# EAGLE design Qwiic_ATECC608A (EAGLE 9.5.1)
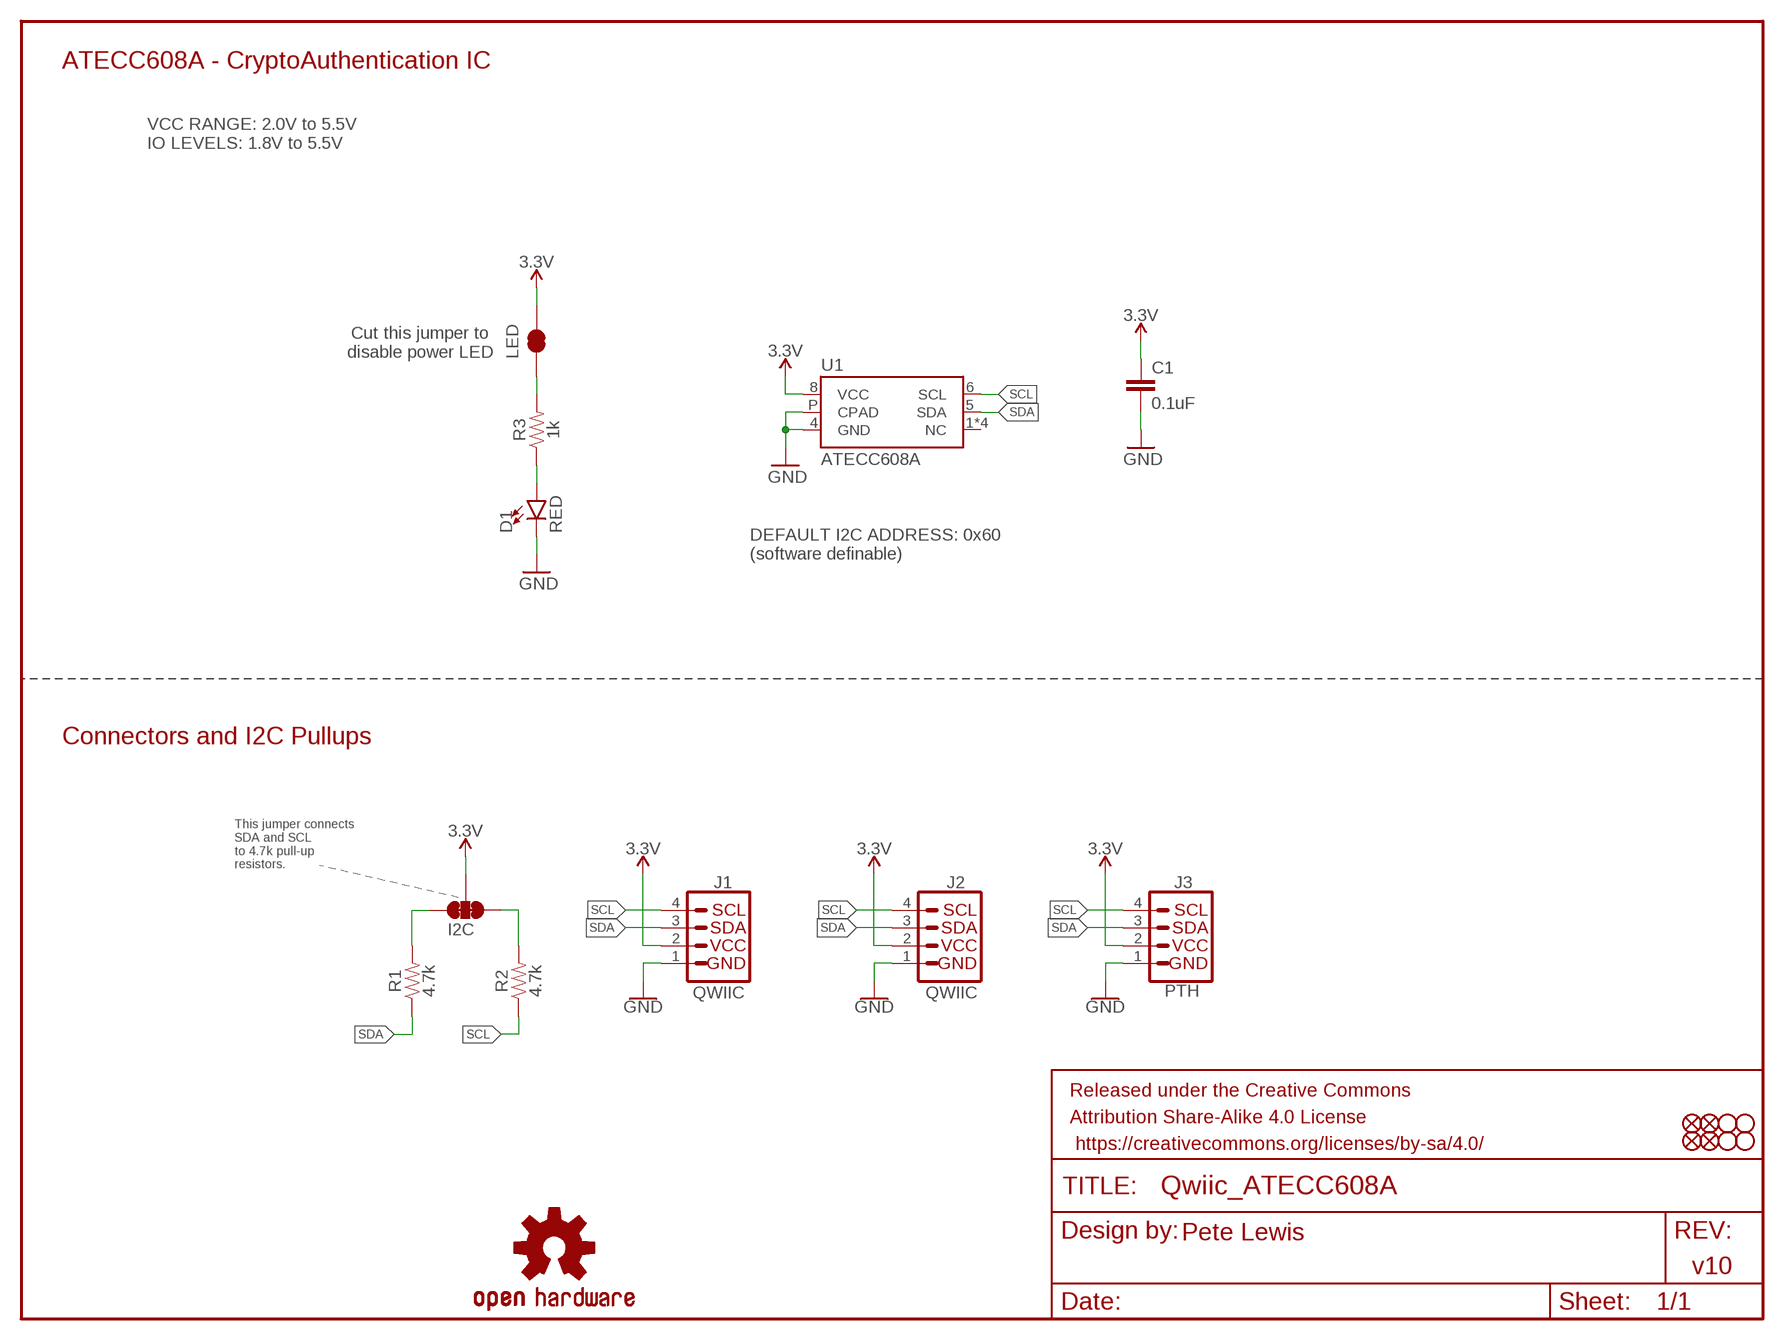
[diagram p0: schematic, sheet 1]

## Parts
C1  0.1uF  0.1UF-0603-25V-(+80/-20%)  [0603]
D1  RED  LED-RED0603  [LED-0603]
FD1  FIDUCIAL1X2  [FIDUCIAL-1X2]
FD2  FIDUCIAL1X2  [FIDUCIAL-1X2]
FD3  FIDUCIAL1X2  [FIDUCIAL-1X2]
FD4  FIDUCIAL1X2  [FIDUCIAL-1X2]
FRAME1  FRAME-LETTER  [CREATIVE_COMMONS]
H1  STAND-OFF  [STAND-OFF]
H2  STAND-OFF  [STAND-OFF]
H3  STAND-OFF  [STAND-OFF]
H4  STAND-OFF  [STAND-OFF]
I2C  JUMPER-SMT_3_2-NC_TRACE_SILK  [SMT-JUMPER_3_2-NC_TRACE_SILK]
J1  QWIIC  I2C_STANDARDQWIIC  [JST04_1MM_RA]
J2  QWIIC  I2C_STANDARDQWIIC  [JST04_1MM_RA]
J3  PTH  I2C_STANDARD_NO_SILK  [1X04_NO_SILK]
LED  JUMPER-SMT_2_NC_TRACE_SILK  [SMT-JUMPER_2_NC_TRACE_SILK]
LOGO4  OSHW-LOGOS  [OSHW-LOGO-S]
R1  4.7k  4.7KOHM-0603-1/10W-1%  [0603]
R2  4.7k  4.7KOHM-0603-1/10W-1%  [0603]
R3  1k  1KOHM-0603-1/10W-1%  [0603]
U1  ATECC608A  ATECC608AUDFN_2X3MM  [UDFN_2X3MM]

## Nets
3.3V: C1.1 I2C.2 J1.2 J2.2 J3.2 LED.2 U1.8(VCC)
GND: C1.2 D1.C J1.1 J2.1 J3.1 U1.4(GND) U1.P(CPAD)
N$3: D1.A R3.1
N$4: I2C.3 R1.2
N$5: I2C.1 R2.2
N$7: LED.1 R3.2
SCL: J1.4 J2.4 J3.4 R2.1 U1.6(SCL)
SDA: J1.3 J2.3 J3.3 R1.1 U1.5(SDA)
Unconnected: U1.1(NC) U1.2(NC) U1.3(NC) U1.7(NC)

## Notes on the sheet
- ATECC608A - CryptoAuthentication IC
- VCC RANGE: 2.0V to 5.5V
  IO LEVELS: 1.8V to 5.5V
- Cut this jumper to 
  disable power LED
- DEFAULT I2C ADDRESS: 0x60
  (software definable)
- Connectors and I2C Pullups
- This jumper connects 
  SDA and SCL 
  to 4.7k pull-up 
  resistors.
- Pete Lewis
- v10

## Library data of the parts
C1 = SparkFun-Capacitors:0.1UF: 0.1µF ceramic capacitors; PROD_ID: CAP-00810
D1 = SparkFun-LED:LED-RED: Red SMD LED; PROD_ID: DIO-00819
FD1-FD4 = SparkFun-Aesthetics:FIDUCIAL: Fiducial Alignment Points
FRAME1 = SparkFun-Aesthetics:FRAME-LETTER: Schematic Frame - Letter
H1-H4 = SparkFun-Hardware:STAND-OFF: Stand Off
I2C = SparkFun-Jumpers:JUMPER-SMT_3_2-NC_TRACE: Normally closed trace jumper (2 of 2 connections) This jumper has a trace between all three pads so they are normally closed (NC). Use a razor knife to open the connection(s). For best results follow the IPC guidelines for cutting traces: Cutout at least 0.063 mm (0.005 in). Remove all loose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
J1 J2 = SparkFun-Connectors:I2C_STANDARD: SparkFun I2C Standard Pinout Header SparkFun has standardized on a pinout for all I2C based sensor breakouts. This pinout allows I2C boards to be plugged directly into the headers on Arduino Uno compatible boards, and to be daisy chained easily. Example SparkFun Products: SparkFun Atmospheric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; PROD_ID: CONN-13694; VALUE: Qwiic Right Angle
J3 = SparkFun-Connectors:I2C_STANDARD: SparkFun I2C Standard Pinout Header SparkFun has standardized on a pinout for all I2C based sensor breakouts. This pinout allows I2C boards to be plugged directly into the headers on Arduino Uno compatible boards, and to be daisy chained easily. Example SparkFun Products: SparkFun Atmospheric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
LED = SparkFun-Jumpers:JUMPER-SMT_2_NC_TRACE: Normally closed trace jumper
LOGO4 = SparkFun-Aesthetics:OSHW-LOGO: Open-Source Hardware (OSHW) Logo
R1 R2 = SparkFun-Resistors:4.7KOHM: 4.7kΩ resistor; PROD_ID: RES-07857
R3 = SparkFun-Resistors:1KOHM: 1kΩ resistor; PROD_ID: RES-07856
U1 = ATECC608A:ATECC608A: ATECC608A CryptoAuthentication Device Cryptographic Co-processor with Secure Hardware-Based Key Storage ECDSA: FIPS186-3 Elliptic Curve Digital Signature Algorithm ECDH: FIPS SP800-56A Elliptic Curve Diffie-Hellman Algorithm AES Algorithm for encryption and decryption NIST Standard P256 Elliptic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; PROD_ID: SPX

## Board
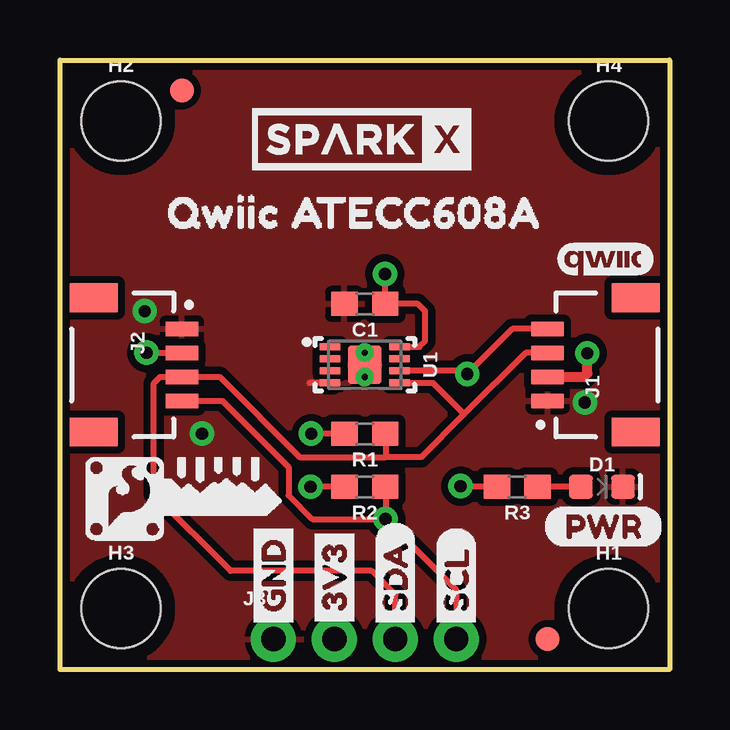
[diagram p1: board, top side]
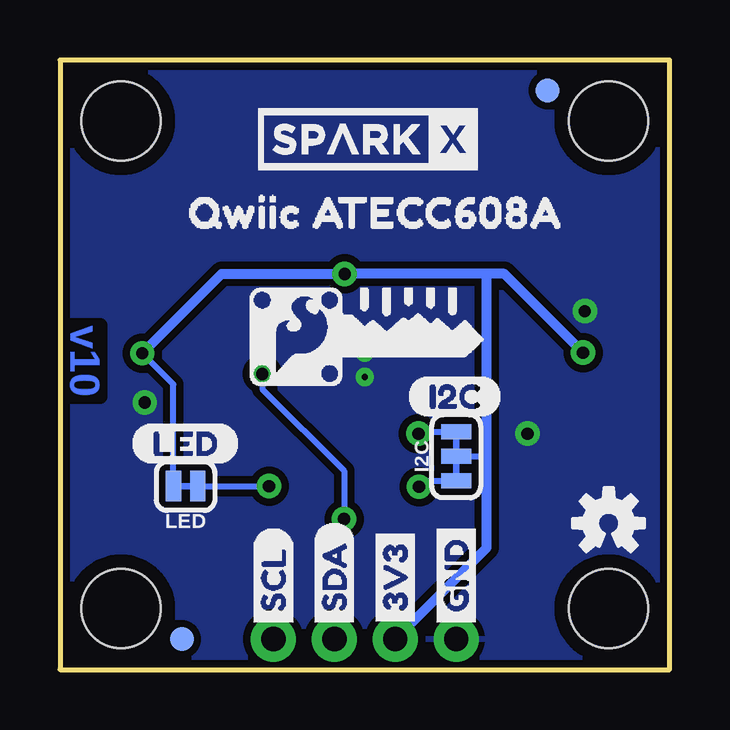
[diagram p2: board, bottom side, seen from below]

Size 25.4 x 25.4 mm. Coordinates in mm from the lower left corner, seen from the top.
Outline: 0,0 0,25.4 25.4,25.4 25.4,0 0,0
Copper layers (1*16): Top 0.035mm / dielectric 1.5mm / Bottom 0.035mm
Design rules "SparkFun-2-layer-STANDARD": minimum track width 10mil, minimum drill 20mil, track to track 10mil, track to pad 8mil, pad to pad 8mil, via to via 10mil, smd to smd 8mil, copper to edge 8mil, drill to drill 8mil, minimum pad ring 10mil, minimum via ring 10mil, stop-mask expansion 4mil, vias tented up to drill 25mil, thermal gap 10mil
tRestrict: area 11,11.8 to 11.4,11.8

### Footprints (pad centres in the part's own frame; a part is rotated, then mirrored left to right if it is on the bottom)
0603 = smd 1.1 x 1: 1 -0.85,0; 2 0.85,0
LED-0603 = smd 1 x 1: A -0.877,0; C 0.877,0
FIDUCIAL-1X2 = smd 1 x 1: 1 0,0
STAND-OFF = hole 3.302: 0,0
SMT-JUMPER_3_2-NC_TRACE_SILK = smd 0.635 x 1.27: 1 -1.016,0; 2 0,0; 3 1.016,0
JST04_1MM_RA = smd 0.6 x 1.35: 1 -1.5,0; 2 -0.5,0; 3 0.5,0; 4 1.5,0 | smd 1.2 x 2: NC1 2.8,-3.675; NC2 -2.8,-3.675
1X04_NO_SILK = drill 1.016 pad 1.88: 1 0,0; 2 2.54,0; 3 5.08,0; 4 7.62,0
SMT-JUMPER_2_NC_TRACE_SILK = smd 0.635 x 1.27: 1 -0.508,0; 2 0.508,0
UDFN_2X3MM = smd 0.3 x 0.85: 1 -0.75,-1.45; 2 -0.25,-1.45; 3 0.25,-1.45; 4 0.75,-1.45; 5 0.75,1.45; 6 0.25,1.45; 7 -0.25,1.45; 8 -0.75,1.45 | smd 1.6 x 1.4: P 0,0

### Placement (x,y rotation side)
C1  12.7,15.24 180 top
D1  22.58,7.62 0 top
FD1  5.08,24.13 0 top
FD2  20.32,1.27 0 top
FD3  20.32,1.27 0 bottom
FD4  5.08,24.13 0 bottom
FRAME1  not placed on the board
H1  22.86,2.54 0 top
H2  2.54,22.86 0 top
H3  2.54,2.54 0 top
H4  22.86,22.86 0 top
I2C  8.89,8.89 90 bottom
J1  20.32,12.7 90 top
J2  5.08,12.7 270 top
J3  8.89,1.27 0 top
LED  20.17,7.65 180 bottom
LOGO4  2.54,6.1 0 bottom
R1  12.7,9.83 180 top
R2  12.7,7.62 180 top
R3  19.05,7.62 180 top
U1  12.7,12.7 270 top
U$1  [LED0]  22.48,9.42 0 bottom
U$2  [3V34]  11.43,1.5 90 top
U$3  [SDA5]  13.97,1.5 90 bottom
U$4  [GND3]  8.89,1.5 90 top
U$5  [SDA5]  13.97,1.5 90 top
U$6  [SCL6]  16.51,1.5 90 top
U$7  [3V34]  11.43,1.5 90 bottom
U$8  [GND3]  8.89,1.5 90 bottom
U$9  [SPARKX-MEDIUM]  12.57,22.1 0 bottom
U$10  [SCL6]  16.51,1.5 90 bottom
U$11  [QWIIC_ATECC608A0]  3.3,19.05 0 top
U$12  [QWIIC_ATECC608A0]  21.21,19.05 0 bottom
U$13  [PWR0]  20.14,5.97 0 top
U$15  [CRYPTO_COPROCESSOR_LOGO#04#PNG]  12.7,13.97 0 bottom
U$16  [QWIIC_4MM]  22.73,17.09 0 top
U$18  [CRYPTO_COPROCESSOR_LOGO#04#PNG]  5.08,7.21 0 top
U$19  [SPARKX-MEDIUM]  12.57,22.1 0 top
U$22  [I2C0]  10.97,11.38 0 bottom

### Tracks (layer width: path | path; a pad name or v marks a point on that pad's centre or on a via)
3.3V  (via drill 0.51)
  Top 0.254: v3.61,13.21 v3.62,13.2 J2.2 | U1.8 14.97,13.45 15.21,13.69 15.21,14.94 14.91,15.24 C1.1 v13.55,16.47 v13.54,16.48
  Top 0.406: J1.2 21.83,12.2 21.97,12.34 v21.97,13.18
  Bottom 0.254: LED.2 20.68,11.89 v21.97,13.18 | I2C.2 7.62,8.89
  Bottom 0.406: 7.62,16.48 6.88,16.48 v3.61,13.21 | 7.62,16.48 v13.54,16.48 18.67,16.48 v21.97,13.18 | J3.2 7.62,5.08 7.62,8.89 7.62,16.48
GND  (via drill 0.25, 0.51)
  Top 0.254: U1.4 10.4,11.95
  other vias: 21.87,11.13 3.53,14.94 12.7,13.21 12.7,12.19 5.92,9.83
  pour Top (isolate 0.305): 0,0 25.4,0 25.4,25.4 0,25.4
  pour Bottom (isolate 0.305): 0,25.4 25.4,25.4 25.4,0 0,0
N$3
  Top 0.254: D1.A R3.1
N$4  (via drill 0.51)
  Top 0.254: R1.2 v10.46,9.83
  Bottom 0.254: v10.46,9.83 10.39,9.91 I2C.3
N$5  (via drill 0.51)
  Top 0.254: R2.2 v10.44,7.62
  Bottom 0.254: v10.44,7.62 10.19,7.87 I2C.1
N$7  (via drill 0.51)
  Top 0.254: v16.69,7.64 18.18,7.64 R3.2
  Bottom 0.254: LED.1 v16.69,7.64
SCL  (via drill 0.51)
  Top 0.254: J1.4 18.85,14.2 v16.97,12.32 16.84,12.45 U1.6 | J2.4 6.76,11.2 9.53,8.43 9.53,7.26 10.52,6.27 v13.56,6.27 | R2.1 13.56,7.61 v13.56,6.27 | v13.56,6.27 16.51,3.33 J3.4
  Bottom 0.254: v13.56,6.27 13.56,8.28 16.97,11.68 v16.97,12.32
SDA
  Top 0.254: J1.3 19.4,13.2 16.83,10.63 | J3.3 13.97,3.12 12.98,4.12 7.11,4.12 3.91,7.32 3.91,11.94 4.17,12.2 J2.3 6.65,12.2 9.99,8.85 13.56,8.85 | R1.1 13.56,9.82 13.56,8.85 | 16.83,10.63 15.05,8.85 13.56,8.85 | U1.5 15.53,11.95 16.83,10.65 16.83,10.63

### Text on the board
Bottom: v10
tDocu: Pete Lewis

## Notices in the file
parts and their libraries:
SparkFun-Aesthetics: Licensing: Creative Commons ShareAlike 4.0 International - https://creativecommons.org/licenses/by-sa/4.0
SparkFun-Aesthetics: Released under the Creative Commons Attribution Share-Alike 4.0 License
SparkFun-Aesthetics: https://creativecommons.org/licenses/by-sa/4.0
